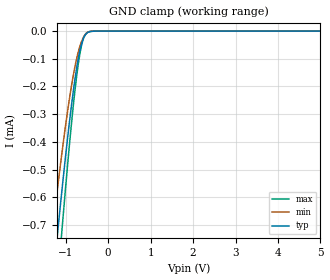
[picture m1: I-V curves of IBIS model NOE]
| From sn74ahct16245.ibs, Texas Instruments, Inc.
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[Model]   NOE
Model_type  Input
Vinl=0.8
Vinh=2.0
| variable   typ   min   max
C_comp   0.83pF   0.74pF   0.94pF
[Temperature Range]   40   100   -40
| Ambient temperature   25   85   -40
[Voltage range]   5   4.5   5.5
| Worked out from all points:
|   GND clamp passes 1 mA (typ) near -1.36 V on its own axis
[GND Clamp]
| NOE
|   Voltage   I(typ)   I(min)   I(max)
-5V       -7.949mA   -6.666mA   -9.002mA
-1.315V   -924.4uA   -726.5uA   -1.15mA
-1.19V    -728.2uA   -564.9uA   -909.7uA
-1.095V   -584.9uA   -448uA     -732.4uA
-1.075V   -555.4uA   -424.2uA   -695.8uA
-885mV    -294.6uA   -218.1uA   -367.8uA
-795mV    -188.2uA   -138.8uA   -232.7uA
-720mV    -113.1uA   -85.43uA   -137.5uA
-655mV    -62.21uA   -49.99uA   -73.29uA
-605mV    -34.6uA    -29.7uA    -38.71uA
-475mV    -4.507uA   -3.732uA   -3.661uA
5V        7.166nA    474.1pA    66.12nA
